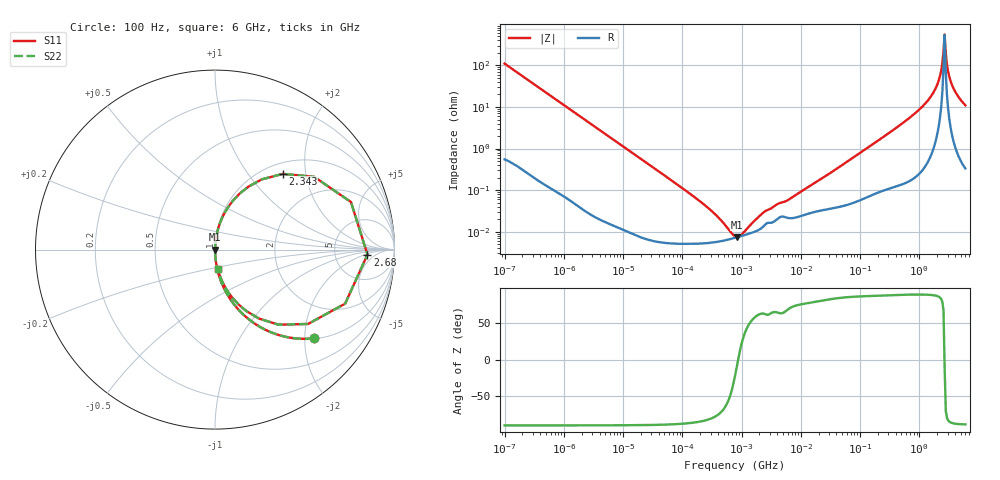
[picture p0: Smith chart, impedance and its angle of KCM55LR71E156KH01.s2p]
!Murata Part Number: KCM55LR71E156KH01
!These Parameters are Measured in Series Mode Connection
!Data Generated on Mar 13, 2026
!  o--ll--o
!Port1  Port2
!  o------o
!Operation Temp=25[degC], DC Bias Voltage=0[V]
!Freq. Start=100[Hz] Stop=6[GHz] 401[Steps]
# Hz S RI R 50
!Freq.(Hz) S11(Real) S11(Imag) S21(Real) S21(Imag) S12(Real) S12(Imag) S22(Real) S22(Imag)
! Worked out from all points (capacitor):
!   401 points, 100 Hz to 6 GHz, reference 50 ohm
!   read as one part in series: C = 14.4 uF near 109 Hz
!   lowest |Z| = 7.44 mohm at 847.2 kHz (marker M1)
!   series resonance near 876.8 kHz, so ESL is about 2.3 nH
!   S11 on the Smith chart (normalised r, x): 100 Hz: 1.01, -2.21; 2.343 GHz: 1.20, +1.49; 2.68 GHz: 12, -2; 6 GHz: 1.01, -0.22
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100  0.55 -0.495  0.45 0.495  0.45 0.495  0.55 -0.495
335  0.1005 -0.2979  0.8995 0.2979  0.8995 0.2979  0.1005 -0.2979
2008  0.00345 -0.0555  0.9966 0.0555  0.9966 0.0555  0.00345 -0.0555
40335  6.4e-05 -0.0028  0.9999 0.0028  0.9999 0.0028  6.4e-05 -0.0028
252896  5.32e-05 -0.000405  0.9999 0.000405  0.9999 0.000405  5.32e-05 -0.000405
619225  6.56e-05 -8.65e-05  0.9999 8.65e-05  0.9999 8.65e-05  6.56e-05 -8.65e-05
774597  7.14e-05 -2.97e-05  0.9999 2.97e-05  0.9999 2.97e-05  7.14e-05 -2.97e-05
847162  7.4e-05 -8.1e-06  0.9999 8.1e-06  0.9999 8.1e-06  7.4e-05 -8.1e-06
1108252  8.27e-05 5.5e-05  0.9999 -5.5e-05  0.9999 -5.5e-05  8.27e-05 5.5e-05
2481164  0.000146 0.000273  0.9999 -0.000273  0.9999 -0.000273  0.000146 0.000273
1.555665e7  0.00029 0.00133  0.9997 -0.00133  0.9997 -0.00133  0.00029 0.00133
3.124326e8  0.00166 0.0239  0.9983 -0.0239  0.9983 -0.0239  0.00166 0.0239
9.150511e8  0.00813 0.0767  0.9919 -0.0767  0.9919 -0.0767  0.00813 0.0767
1.637704e9  0.0439 0.1857  0.9561 -0.1857  0.9561 -0.1857  0.0439 0.1857
2.048624e9  0.1371 0.3115  0.8629 -0.3115  0.8629 -0.3115  0.1371 0.3115
2.34314e9  0.3782 0.422  0.6218 -0.422  0.6218 -0.422  0.3782 0.422
2.450438e9  0.553 0.4052  0.447 -0.4052  0.447 -0.4052  0.553 0.4052
2.679998e9  0.8495 -0.0277  0.1505 0.0277  0.1505 0.0277  0.8495 -0.0277
2.931063e9  0.5189 -0.4142  0.4811 0.4142  0.4811 0.4142  0.5189 -0.4142
3.065283e9  0.3539 -0.4184  0.6461 0.4184  0.6461 0.4184  0.3539 -0.4184
3.666503e9  0.0995 -0.2716  0.9005 0.2716  0.9005 0.2716  0.0995 -0.2716
6e9  0.0151 -0.1075  0.9849 0.1075  0.9849 0.1075  0.0151 -0.1075
